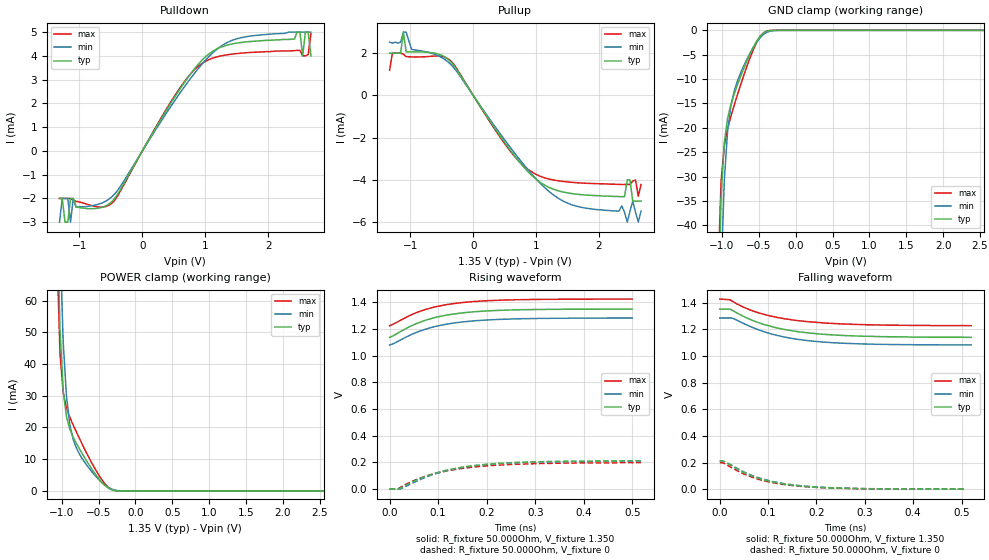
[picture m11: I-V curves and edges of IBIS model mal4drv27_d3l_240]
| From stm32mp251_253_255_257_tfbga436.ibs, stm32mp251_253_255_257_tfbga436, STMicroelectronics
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[Model] mal4drv27_d3l_240
Model_type   I/O
Polarity   Non-Inverting
Enable   Active-High
C_comp   1.684pF   1.663pF   1.711pF
C_comp_pullup   812.334fF   800.254fF   826.800fF
C_comp_pulldown   769.496fF   756.297fF   787.425fF
Vinh = 805.000mV
Vinl = 545.000mV
Vmeas = 675.000mV
Vref = 675.000mV
Rref = 50Ohms
Cref = 0pF
[Model Spec]
Vinh   805.000mV   772.000mV   855.000mV
Vinl   545.000mV   512.000mV   595.000mV
Vmeas   675.000mV   642.000mV   725.000mV
Vref   675.000mV   642.000mV   725.000mV
D_overshoot_ampl_h 0.4 NA   NA
D_overshoot_ampl_l 0.4 NA   NA
D_overshoot_area_l 110.000m NA   NA
D_overshoot_area_h 110.000m NA   NA
[Temperature Range]   25.000   125.000   -40.000
[Voltage Range]   1.350V   1.283V   1.425V
[GND Clamp Reference]   0.00V   0.00V   0.00V
[C Comp Corner]
| variable   typ   min   max
C_comp   1.684pF   1.663pF   1.711pF
C_comp_pullup   812.334fF   800.254fF   826.800fF
C_comp_pulldown   769.496fF   756.297fF   787.425fF
[Pulldown Reference]   0.00V   0.00V   0.00V
[POWER Clamp Reference]   1.350V   1.283V   1.425V
[Pullup Reference]   1.350V   1.283V   1.425V
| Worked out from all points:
|   slope of the pulldown table from 0 to 0.203 V, typ, clamps not added: 220 ohm
|   slope of the pullup table from 0 to 0.203 V, typ, clamps not added: 218 ohm
|   GND clamp passes 1 mA (typ) near -0.47 V on its own axis
|   POWER clamp passes 1 mA (typ) near -0.37 V on its own axis
|   rising waveform, R_fixture 50.000Ohm, V_fixture 1.350: 20-80 % time 100ps typ, 103ps min, 99ps max; typ from 1.14 V to 1.35 V
|   rising waveform, R_fixture 50.000Ohm, V_fixture 0: 20-80 % time 120ps typ, 114ps min, 121ps max; typ from 0 V to 0.212 V
|   falling waveform, R_fixture 50.000Ohm, V_fixture 1.350: 20-80 % time 119ps typ, 115ps min, 120ps max; typ from 1.35 V to 1.14 V
|   falling waveform, R_fixture 50.000Ohm, V_fixture 0: 20-80 % time 98.6ps typ, 102ps min, 97.3ps max; typ from 0.213 V to 0 V
[GND Clamp]
-1.318V   -672mA     -638mA     -661.1mA
-1.054V   -60.41mA   -84.99mA   -50.75mA
-1.011V   -34.02mA   -49.92mA   -30.84mA
-966.7mV  -22.91mA   -30.54mA   -23.58mA
-922.7mV  -18.04mA   -20.68mA   -20.16mA
-878.8mV  -15.25mA   -15.56mA   -17.69mA
-834.8mV  -13.14mA   -12.55mA   -15.44mA
-747mV    -9.486mA   -8.743mA   -11.21mA
-615.2mV  -4.709mA   -4.591mA   -5.504mA
-439.4mV  -562.2uA   -889.5uA   -546.1uA
-219.7mV  -954.1nA   -9.356uA   -215nA
2.68V     18.98nA    945nA      23.53nA
[Power Clamp]
-1.33V    889mA      842.2mA    872.8mA
-1.067V   94.44mA    130.9mA    77.96mA
-1.023V   51.04mA    78.45mA    43.53mA
-978.8mV  31.54mA    46.94mA    31.01mA
-934.8mV  23.45mA    29.85mA    26.15mA
-890.9mV  19.58mA    21.13mA    23.3mA
-847mV    17.11mA    16.47mA    20.93mA
-671.2mV  9.815mA    8.474mA    12.37mA
-495.5mV  3.823mA    3.529mA    4.955mA
-363.6mV  819.5uA    1.024mA    1.072mA
-187.9mV  4.227uA    28.6uA     2.566uA
2.668V    -29.12nA   -796.8nA   -15.73nA
[Pulldown]
-1.318V   -2mA       -3mA       -2mA
-1.23V    -3mA       -2mA       -2mA
-1.142V   -2mA       -3mA       -2mA
-1.099V   -2mA       -2mA       -2.062mA
-483.3mV  -2.131mA   -1.927mA   -2.2mA
615.2mV   2.672mA    2.498mA    2.716mA
1.142V    4.23mA     4.182mA    3.923mA
2.505V    5mA        5mA        4.23mA
2.549V    4mA        5mA        4mA
2.592V    5mA        5mA        4mA
2.636V    5mA        5mA        4.053mA
2.68V     4mA        5mA        4.931mA
[Pullup]
-1.33V    2mA        2.525mA    1.193mA
-1.155V   2mA        2.526mA    2mA
-1.111V   3mA        3mA        1.955mA
-1.067V   2.07mA     3mA        1.837mA
-407.6mV  1.734mA    1.605mA    1.748mA
690.9mV   -2.988mA   -2.855mA   -3.001mA
1.306V    -4.471mA   -4.776mA   -4.018mA
2.405V    -4.79mA    -5.524mA   -4.213mA
2.492V    -4mA       -5.476mA   -4.217mA
2.536V    -5mA       -5mA       -4.058mA
2.624V    -5mA       -6mA       -4.771mA
2.668V    -5mA       -5.475mA   -4.211mA
[Ramp]
R_load=50.000Ohm
dV/dt_r   126.900mV/111.000ps  123.297mV/109.500ps  119.400mV/112.500ps
dV/dt_f   126.900mV/109.500ps  123.297mV/110.500ps  119.400mV/110.000ps
[Rising waveform]
R_fixture=50.000Ohm
V_fixture=1.350
V_fixture_min=1.283
V_fixture_max=1.425
0s        1.138V     1.081V     1.225V
10ps      1.155V     1.094V     1.241V
44ps      1.223V     1.157V     1.306V
72ps      1.264V     1.197V     1.345V
106ps     1.297V     1.229V     1.376V
127ps     1.31V      1.242V     1.389V
153ps     1.323V     1.255V     1.4V
193ps     1.335V     1.267V     1.411V
272ps     1.345V     1.278V     1.421V
500ps     1.35V      1.283V     1.425V
[Rising waveform]
R_fixture=50.000Ohm
V_fixture=0
0s        -399.9uV   -473.5uV   -65.9uV
18ps      -399.9uV   -473.5uV   4.005mV
21ps      5.084mV    -473.5uV   10.33mV
56ps      70mV       60.56mV    72.84mV
98ps      124mV      119mV      121mV
134ps     154mV      152mV      147mV
172ps     176mV      174mV      165mV
218ps     191mV      190mV      178mV
291ps     204mV      202mV      190mV
518ps     212mV      209mV      198mV
[Falling waveform]
R_fixture=50.000Ohm
V_fixture=1.350
V_fixture_min=1.283
V_fixture_max=1.425
0s        1.351V     1.284V     1.426V
21ps      1.351V     1.284V     1.421V
25ps      1.343V     1.284V     1.412V
63ps      1.273V     1.22V      1.344V
102ps     1.225V     1.17V      1.301V
135ps     1.197V     1.14V      1.278V
187ps     1.17V      1.113V     1.255V
235ps     1.157V     1.098V     1.243V
305ps     1.147V     1.088V     1.233V
520ps     1.139V     1.082V     1.226V
[Falling waveform]
R_fixture=50.000Ohm
V_fixture=0
0s        213mV      210mV      200mV
6ps       213mV      210mV      198mV
14ps      198mV      201mV      184mV
45ps      133mV      139mV      123mV
75ps      87.55mV    92.59mV    79.9mV
108ps     54.8mV     58.81mV    49.61mV
149ps     30.45mV    33.4mV     27.2mV
189ps     17.15mV    19.21mV    15.65mV
254ps     6.704mV    7.746mV    5.957mV
506ps     171uV      218.9uV    123.9uV
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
